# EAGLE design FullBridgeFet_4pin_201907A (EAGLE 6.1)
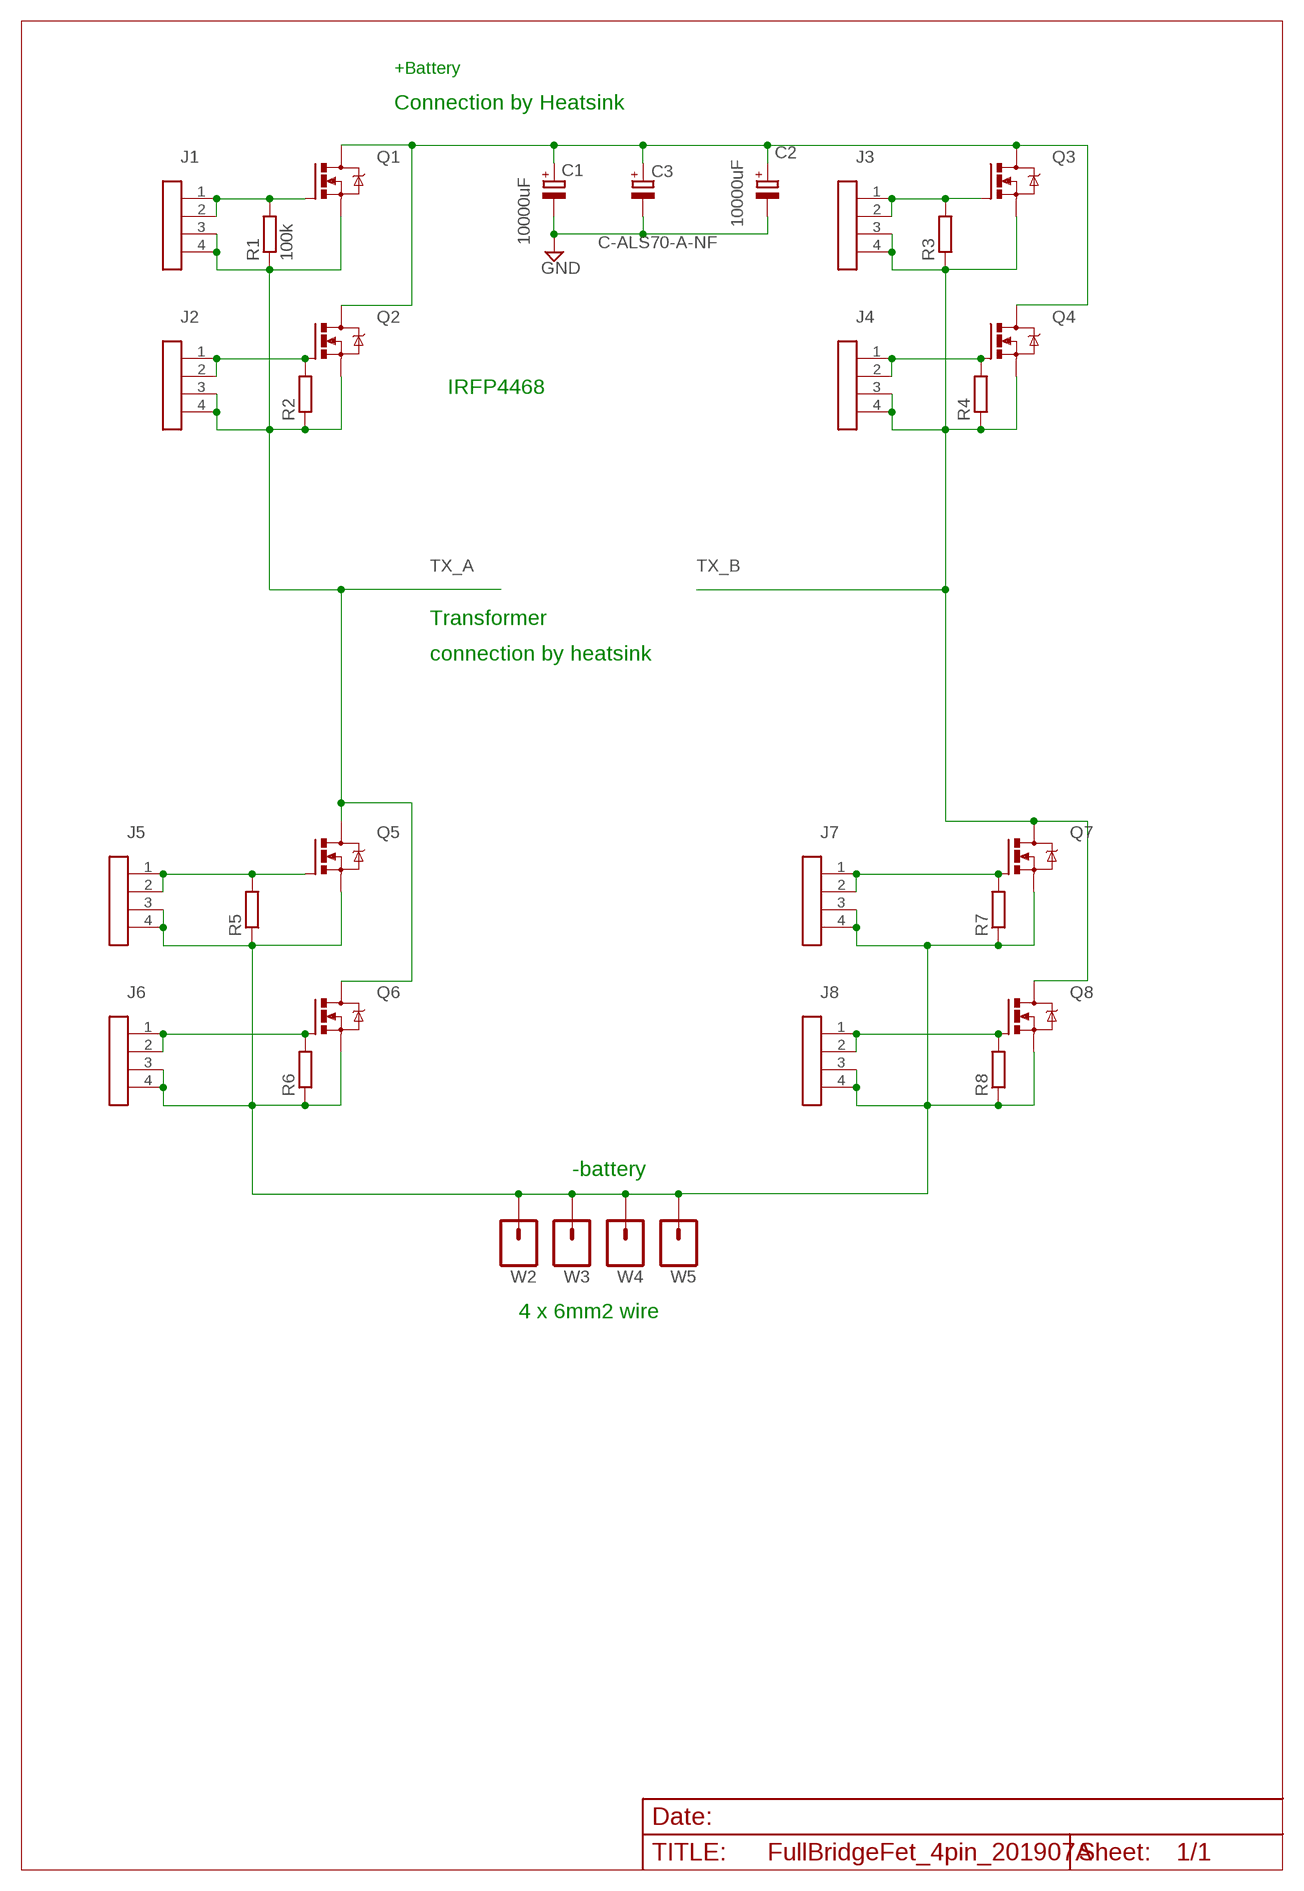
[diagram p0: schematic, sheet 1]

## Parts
C1  10000uF  C-RB3500LARGEPTH  [EB35D_LARGETH]
C2  10000uF  C-RB3500LARGEPTH  [EB35D_LARGETH]
C3  C-ALS70-A-NF  [C-ALS70-A-NF]
J1  IDC04  [IDC04]
J2  IDC04  [IDC04]
J3  IDC04  [IDC04]
J4  IDC04  [IDC04]
J5  IDC04  [IDC04]
J6  IDC04  [IDC04]
J7  IDC04  [IDC04]
J8  IDC04  [IDC04]
Q1  IRFP4468  MOSFET-NCH-BIG  [TO247-WIRED]
Q2  MOSFET-NCH-BIG  [TO247-WIRED]
Q3  MOSFET-NCH-BIG  [TO247-WIRED]
Q4  MOSFET-NCH-BIG  [TO247-WIRED]
Q5  MOSFET-NCH-BIG  [TO247-WIRED]
Q6  MOSFET-NCH-BIG  [TO247-WIRED]
Q7  MOSFET-NCH-BIG  [TO247-WIRED]
Q8  MOSFET-NCH-BIG  [TO247-WIRED]
R1  100k  R-EU_R1206  [R1206]
R2  R-EU_R1206  [R1206]
R3  R-EU_R1206  [R1206]
R4  R-EU_R1206  [R1206]
R5  R-EU_R1206  [R1206]
R6  R-EU_R1206  [R1206]
R7  R-EU_R1206  [R1206]
R8  R-EU_R1206  [R1206]
W2  M014MM2-WIREHOLE  [3.5MMWIREHOLE]
W3  M014MM2-WIREHOLE  [3.5MMWIREHOLE]
W4  M014MM2-WIREHOLE  [3.5MMWIREHOLE]
W5  M014MM2-WIREHOLE  [3.5MMWIREHOLE]

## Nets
+BATT: C1.+ C2.+ C3.POS2(+) C3.POS(+) Q1.D Q1.DW(D) Q2.D Q2.DW(D) Q3.D Q3.DW(D) Q4.D Q4.DW(D)
GND: C1.- C2.- C3.NEG2(-) C3.NEG(-) J5.3 J5.4 J6.3 J6.4 J7.3 J7.4 J8.3 J8.4 Q5.S Q5.SW(S) Q6.S Q6.SW(S) Q7.S Q7.SW(S) Q8.S Q8.SW(S) R5.1 R6.1 R7.1 R8.1 W2.P$1 W3.P$1 W4.P$1 W5.P$1
N$1: J1.1 J1.2 Q1.G R1.2
N$2: J5.1 J5.2 Q5.G R5.2
N$3: J6.1 J6.2 Q6.G R6.2
N$4: J7.1 J7.2 Q7.G R7.2
N$5: J2.1 J2.2 Q2.G R2.2
N$6: J8.1 J8.2 Q8.G R8.2
N$7: J3.1 J3.2 Q3.G R3.2
N$10: J4.1 J4.2 Q4.G R4.2
TX_A: J1.3 J1.4 J2.3 J2.4 Q1.S Q1.SW(S) Q2.S Q2.SW(S) Q5.D Q5.DW(D) Q6.D Q6.DW(D) R1.1 R2.1
TX_B: J3.3 J3.4 J4.3 J4.4 Q3.S Q3.SW(S) Q4.S Q4.SW(S) Q7.D Q7.DW(D) Q8.D Q8.DW(D) R3.1 R4.1

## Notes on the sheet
- +Battery
- Connection by Heatsink
- IRFP4468
- Transformer
- connection by heatsink
- -battery
- 4 x 6mm2 wire

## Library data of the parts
C1 C2 = Andrew Passive:C-RB3500
C3 = Andrew Passive:C-ALS70-A-NF
J1-J8 = Andrew_Connectors:IDC04
Q1-Q8 = Andrew Transistor:MOSFET-NCH-BIG
R1-R8 = resistor:R-EU_: RESISTOR, European symbol
W2-W5 = Andrew:M01: Header 1

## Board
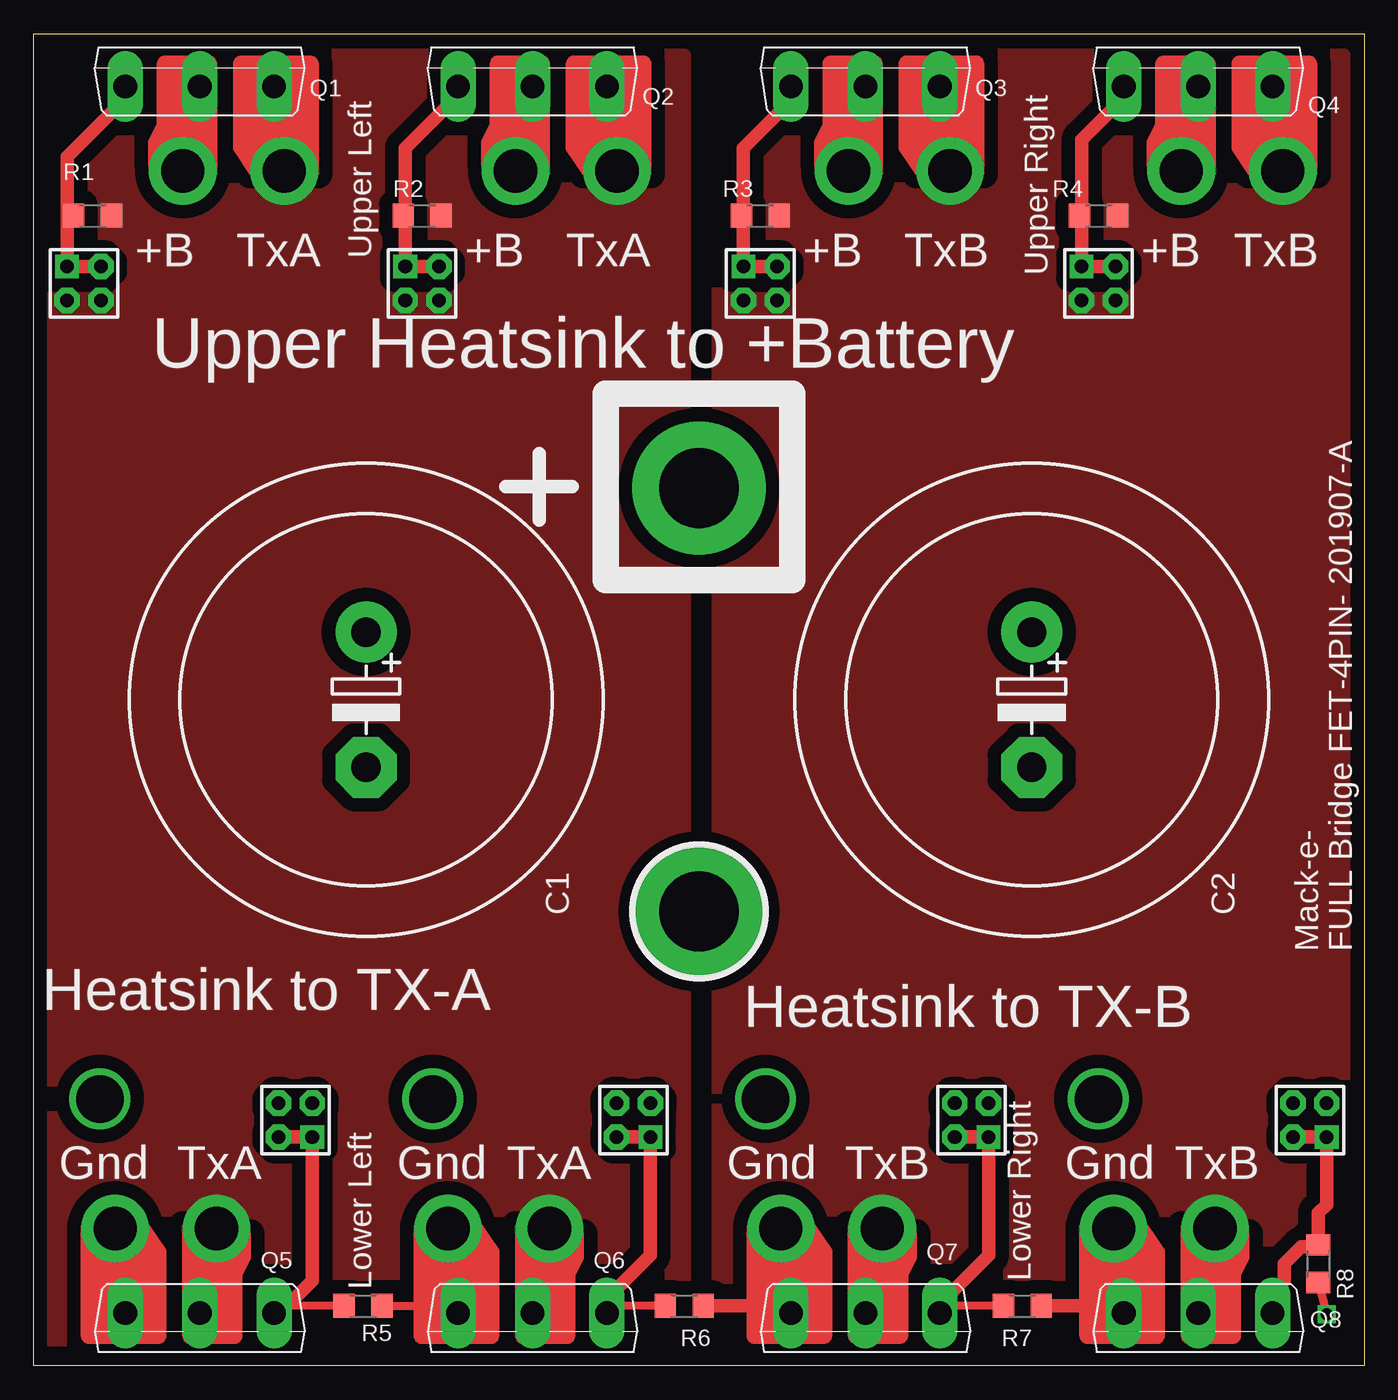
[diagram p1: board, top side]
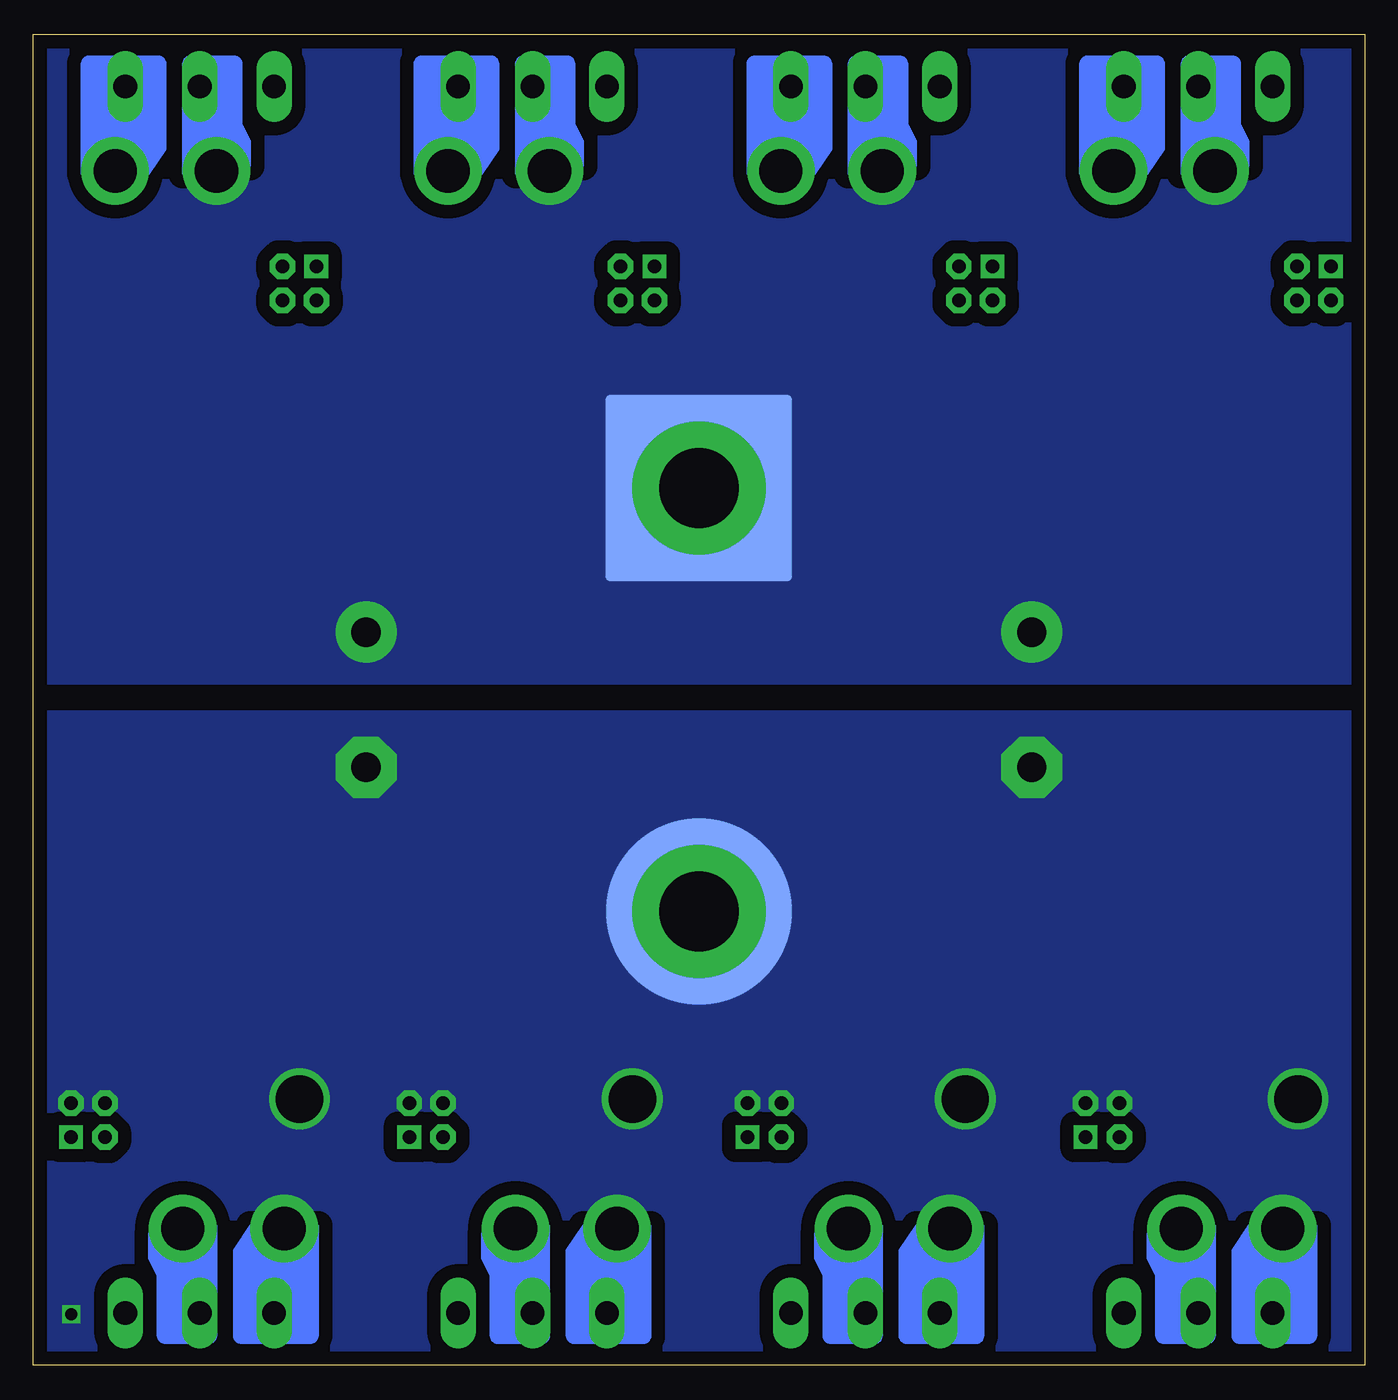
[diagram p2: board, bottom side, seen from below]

Size 100 x 100 mm. Coordinates in mm from the lower left corner, seen from the top.
Outline: 0,0 100,0 100,100 0,100 0,0
Copper layers (1*16): Top 0.035mm / dielectric 1.5mm / Bottom 0.035mm
Design rules: minimum track width 10mil, minimum drill 24mil, track to track 8mil, track to pad 8mil, pad to pad 8mil, via to via 8mil, smd to smd 8mil, copper to edge 40mil, drill to drill 8mil, minimum pad ring 10mil, minimum via ring 8mil, stop-mask expansion 4mil, vias tented up to drill 0mil, thermal gap 10mil

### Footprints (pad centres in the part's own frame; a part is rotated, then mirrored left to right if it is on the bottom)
EB35D_LARGETH = drill 2.2 pad 4.597: + -5.08,0 | drill 2.2 pad 4.597 octagon: - 5.08,0
C-ALS70-A-NF = drill 6 pad 10: NEG 0,-15.9; POS 0,15.9 | smd 14 x 14 bottom: NEG2 0,-15.9; POS2 0,15.9
IDC04 = drill 1.016 pad 1.778 square: 1 -1.27,1.27 | drill 1.016 pad 1.905 octagon: 2 1.27,1.27; 3 -1.27,-1.27; 4 1.27,-1.27
TO247-WIRED = drill 1.778 long: D 0,-2.921; G -5.588,-2.921; S 5.588,-2.921 | drill 3.25 pad 5.08: DW -1.27,-9.271; SW 6.35,-9.271
R1206 = smd 1.6 x 1.803: 1 -1.422,0; 2 1.422,0
3.5MMWIREHOLE = drill 3.556: P$1 0,0

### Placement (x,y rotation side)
C1  25,50 270 top
C2  75,50 270 top
C3  50,50 0 top
J1  3.81,81.28 0 top
J2  29.21,81.28 0 top
J3  54.61,81.28 0 top
J4  80.01,81.28 0 top
J5  19.68,18.41 180 top
J6  45.09,18.41 180 top
J7  70.48,18.41 180 top
J8  95.89,18.41 180 top
Q1  12.5,99 0 top
Q2  37.5,99 0 top
Q3  62.5,99 0 top
Q4  87.5,99 0 top
Q5  12.5,1 180 top
Q6  37.5,1 180 top
Q7  62.5,1 180 top
Q8  87.5,1 180 top
R1  4.45,86.36 180 top
R2  29.21,86.36 180 top
R3  54.61,86.36 180 top
R4  80.01,86.36 180 top
R5  24.77,4.45 180 top
R6  48.9,4.45 180 top
R7  74.3,4.45 180 top
R8  96.52,7.62 90 top
W2  80,20 0 top
W3  55,20 0 top
W4  30,20 0 top
W5  5,20 0 top

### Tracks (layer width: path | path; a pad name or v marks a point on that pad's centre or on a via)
+BATT
  pour Bottom (isolate 1.016, no thermals): 0.64,52.07 0.64,99.06 99.06,99.06 99.06,51.44 0.64,51.44
GND  (via drill 0.9)
  Top 0.61: 81.91,4.45 Q8.S | Q7.S 56.91,4.45 57.15,4.45 57.15,3.81 | R5.1 31.91,4.45 Q6.S | R8.1 v97.16,3.81
  Top 1.016: R6.1 56.91,4.45 | R7.1 81.91,4.45
  pour Bottom (isolate 1.016, no thermals): 0.64,48.9 99.06,48.9 99.06,1.27 0.64,1.27
N$1
  Top 0.406: R1.2 2.54,86.36
  Top 1.016: Q1.G 6.91,95.18 2.54,90.81 2.54,86.36 J1.1 J1.2
N$2
  Top 0.61: R5.2 18.09,4.45 Q5.G
  Top 1.016: Q5.G 18.53,3.92 20.95,6.35 J5.1 J5.2
N$3
  Top 0.61: R6.2 43.09,4.45 Q6.G
  Top 1.016: Q6.G 43.09,4.99 46.35,8.26 J6.1 J6.2
N$4
  Top 0.61: R7.2 68.09,4.45
  Top 1.016: Q7.G 68.09,4.45 68.09,4.59 71.75,8.26 J7.1 J7.2
N$5
  Top 0.406: R2.2 27.94,86.36
  Top 1.016: Q2.G 31.91,95.41 27.94,91.44 27.94,86.36 J2.1 J2.2
N$6
  Top 1.016: 95.89,8.89 95.25,8.89 93.98,7.62 93.98,6.35 93.09,5.46 Q8.G | 95.89,8.89 96.52,8.89 | 95.89,8.89 96.04,9.04 R8.2 96.52,11.43 97.16,12.06 J8.1 J8.2
N$7
  Top 0.61: R3.2 53.34,86.36
  Top 1.016: Q3.G 56.91,95.01 53.34,91.44 53.34,86.36 J3.1 J3.2
N$10
  Top 0.61: R4.2 78.74,86.36
  Top 1.016: Q4.G 81.91,95.25 78.74,92.08 78.74,86.36 J4.1 J4.2
TX_A
  pour Top (isolate 1.016, no thermals): 1.27,98.42 48.26,98.42 48.9,98.42 48.9,1.91 1.27,1.91
TX_B
  pour Top (isolate 1.016, no thermals): 51.44,98.42 98.42,98.42 98.42,1.91 51.44,1.91

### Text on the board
tPlace: +B | TxA | Upper Left | +B | TxA | +B | TxB | +B | TxB | Upper Right | Upper Heatsink to +Battery | Mack-e- | FULL Bridge FET-4PIN- 201907-A | Heatsink to TX-A | Heatsink to TX-B | Gnd | TxA | Gnd | TxA | Gnd | TxB | Gnd | TxB | Lower Left | Lower Right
